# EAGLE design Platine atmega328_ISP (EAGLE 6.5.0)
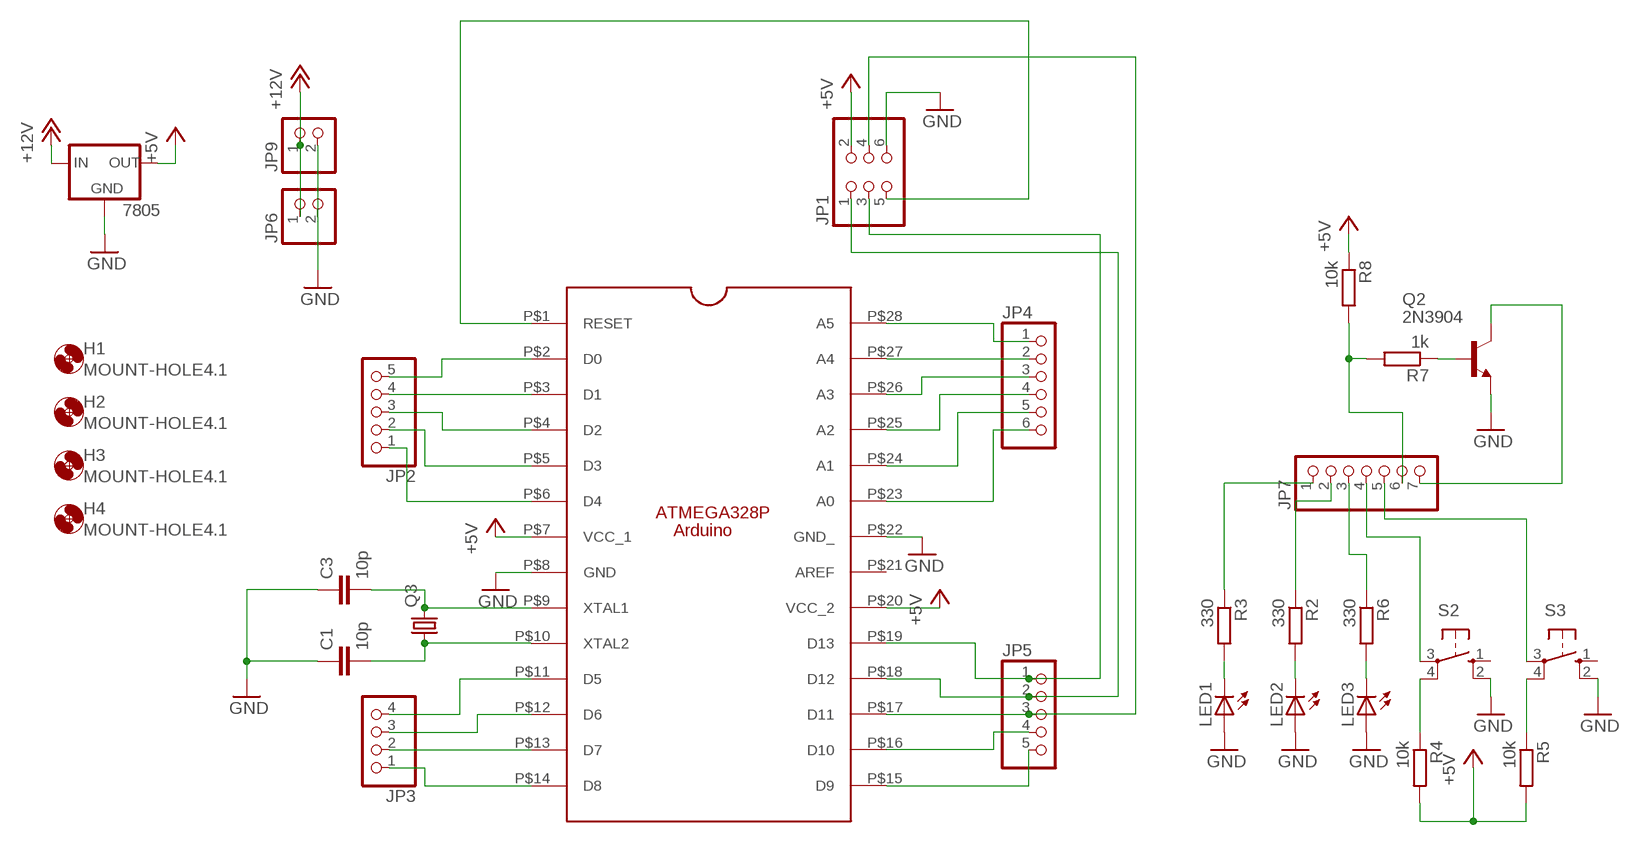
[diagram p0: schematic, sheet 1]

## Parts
7805  78LXX  [78LXX]
C1  10p  C-EU050-025X075  [C050-025X075]
C3  10p  C-EU050-025X075  [C050-025X075]
H1  MOUNT-HOLE4.1  [4,1]
H2  MOUNT-HOLE4.1  [4,1]
H3  MOUNT-HOLE4.1  [4,1]
H4  MOUNT-HOLE4.1  [4,1]
JP1  PINHD-2X3/OCT  [2X03]
JP2  PINHD-1X5  [1X05]
JP3  PINHD-1X4  [1X04]
JP4  PINHD-1X6  [1X06]
JP5  PINHD-1X5  [1X05]
JP6  PINHD-1X2  [1X02]
JP7  PINHD-1X7  [1X07]
JP9  PINHD-1X2  [1X02]
LED1  LED3MM  [LED3MM]
LED2  LED3MM  [LED3MM]
LED3  LED3MM  [LED3MM]
Q2  2N3904  [TO92]
Q3  CRYSTALHC49S  [HC49/S]
R2  330  R-EU_0207/7  [0207/7]
R3  330  R-EU_0207/7  [0207/7]
R4  10k  R-EU_0207/7  [0207/7]
R5  10k  R-EU_0207/7  [0207/7]
R6  330  R-EU_0207/7  [0207/7]
R7  1k  R-EU_0207/7  [0207/7]
R8  10k  R-EU_0207/7  [0207/7]
S2  10-XX  [B3F-10XX]
S3  10-XX  [B3F-10XX]
U1  ATMEGA328P  [ATMEGA328P]

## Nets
7805: 7805.OUT ; supply symbol labelled +5V
+5V: JP1.2 R4.2 R5.2 R8.1 U1.P$7(VCC_1) U1.P$20(VCC_2)
+12V: 7805.IN JP6.1 JP9.1
GND: 7805.GND C1.1 C3.1 JP1.6 JP9.2 LED1.A LED2.A LED3.A Q2.3(E) S2.2(S1) S3.2(S1) U1.P$8(GND) U1.P$22(GND_)
N$1: C3.2 Q3.2 U1.P$9(XTAL1)
N$2: C1.2 Q3.1 U1.P$10(XTAL2)
N$3: JP1.5 U1.P$1(RESET)
N$4: JP2.5 U1.P$2(D0)
N$5: JP2.4 U1.P$3(D1)
N$6: JP2.3 U1.P$4(D2)
N$7: JP2.2 U1.P$5(D3)
N$8: JP2.1 U1.P$6(D4)
N$9: JP5.5 U1.P$15(D9)
N$10: JP5.4 U1.P$16(D10)
N$11: JP1.4 JP5.3 U1.P$17(D11)
N$12: JP1.1 JP5.2 U1.P$18(D12)
N$13: JP1.3 JP5.1 U1.P$19(D13)
N$14: JP4.1 U1.P$28(A5)
N$15: JP4.2 U1.P$27(A4)
N$16: JP4.3 U1.P$26(A3)
N$17: JP4.4 U1.P$25(A2)
N$18: JP4.5 U1.P$24(A1)
N$19: JP4.6 U1.P$23(A0)
N$20: LED1.K(C) R3.2
N$21: R4.1 S2.4(P1)
N$22: JP7.7 Q2.1(C)
N$23: R5.1 S3.4(P1)
N$24: JP7.1 R3.1
N$25: LED2.K(C) R2.2
N$26: LED3.K(C) R6.2
N$27: JP7.2 R2.1
N$28: JP7.3 R6.1
N$29: JP7.4 S2.3(P)
N$30: JP7.5 S3.3(P)
N$31: JP7.6 R7.2 R8.2
N$32: Q2.2(B) R7.1
N$33: JP3.1 U1.P$14(D8)
N$34: JP3.2 U1.P$13(D7)
N$35: JP3.3 U1.P$12(D6)
N$36: JP3.4 U1.P$11(D5)
Unconnected: JP6.2 S2.1(S) S3.1(S) U1.P$21(AREF)

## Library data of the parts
7805 = v-reg:78LXX: VOLTAGE REGULATOR
C1 C3 = rcl:C-EU: CAPACITOR, European symbol
H1-H4 = holes:MOUNT-HOLE: MOUNTING HOLE with drill center marker
JP1 = pinhead_v2:PINHD-2X3: PIN HEADER
JP2 JP5 = pinhead:PINHD-1X5: PIN HEADER
JP3 = pinhead:PINHD-1X4: PIN HEADER
JP4 = pinhead:PINHD-1X6: PIN HEADER
JP6 JP9 = pinhead:PINHD-1X2: PIN HEADER
JP7 = pinhead:PINHD-1X7: PIN HEADER
LED1-LED3 = led:LED: LED
Q2 = transistor-npn:2N3904: NPN Transistor
Q3 = crystal:CRYSTAL: CRYSTAL
R2-R8 = rcl:R-EU_: RESISTOR, European symbol
S2 S3 = switch-omron:10-XX: OMRON SWITCH; MPN: B3F-1000; OC_FARNELL: 176432; OC_NEWARK: 36M3542
U1 = Atmega328P:ATMEGA328P

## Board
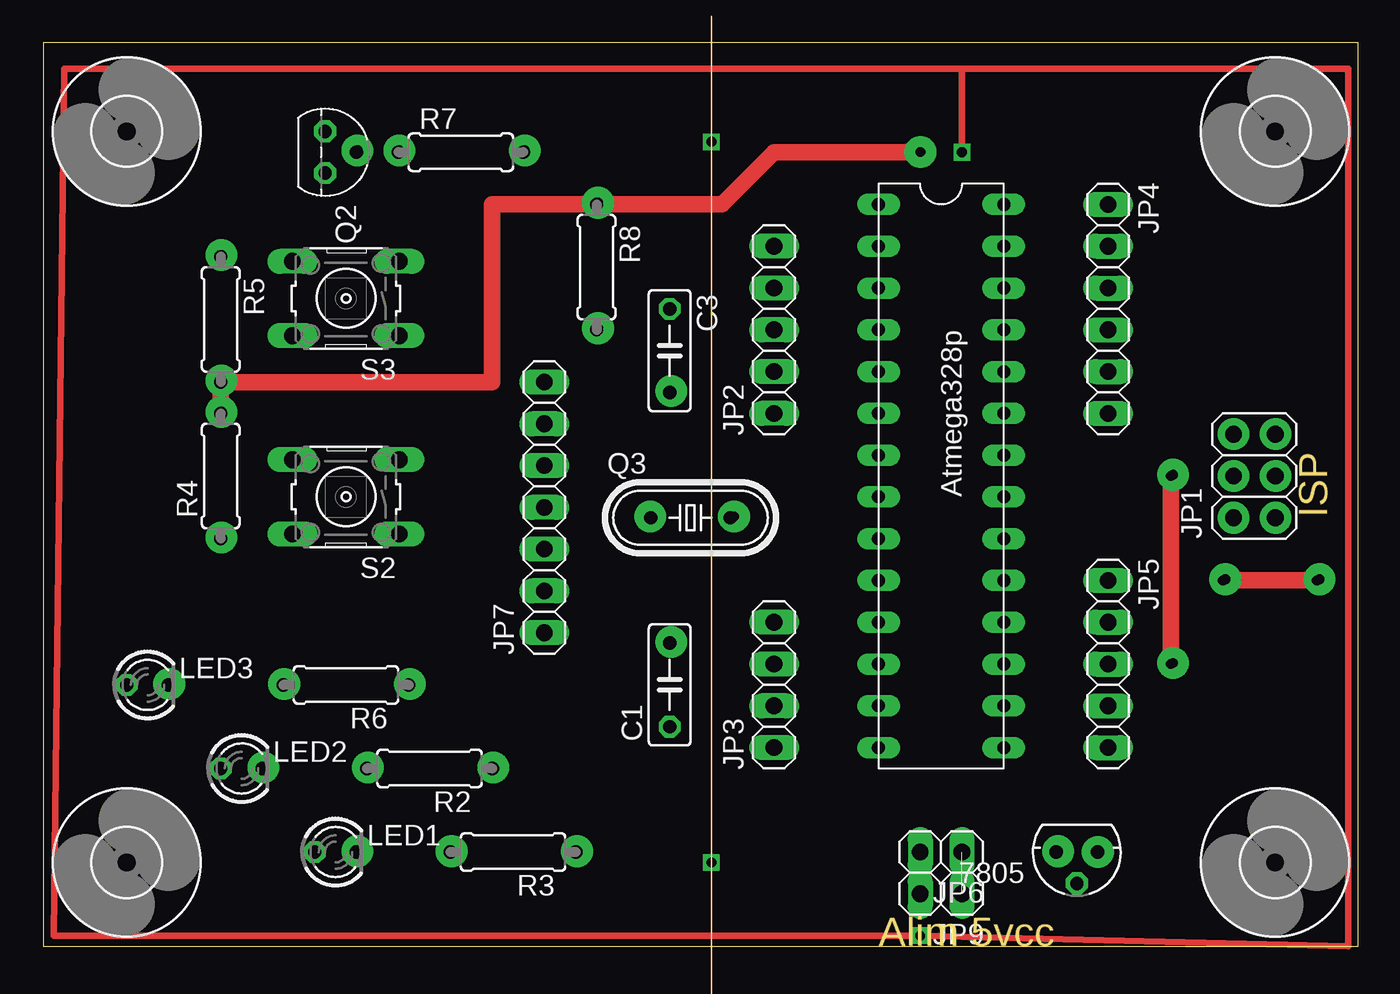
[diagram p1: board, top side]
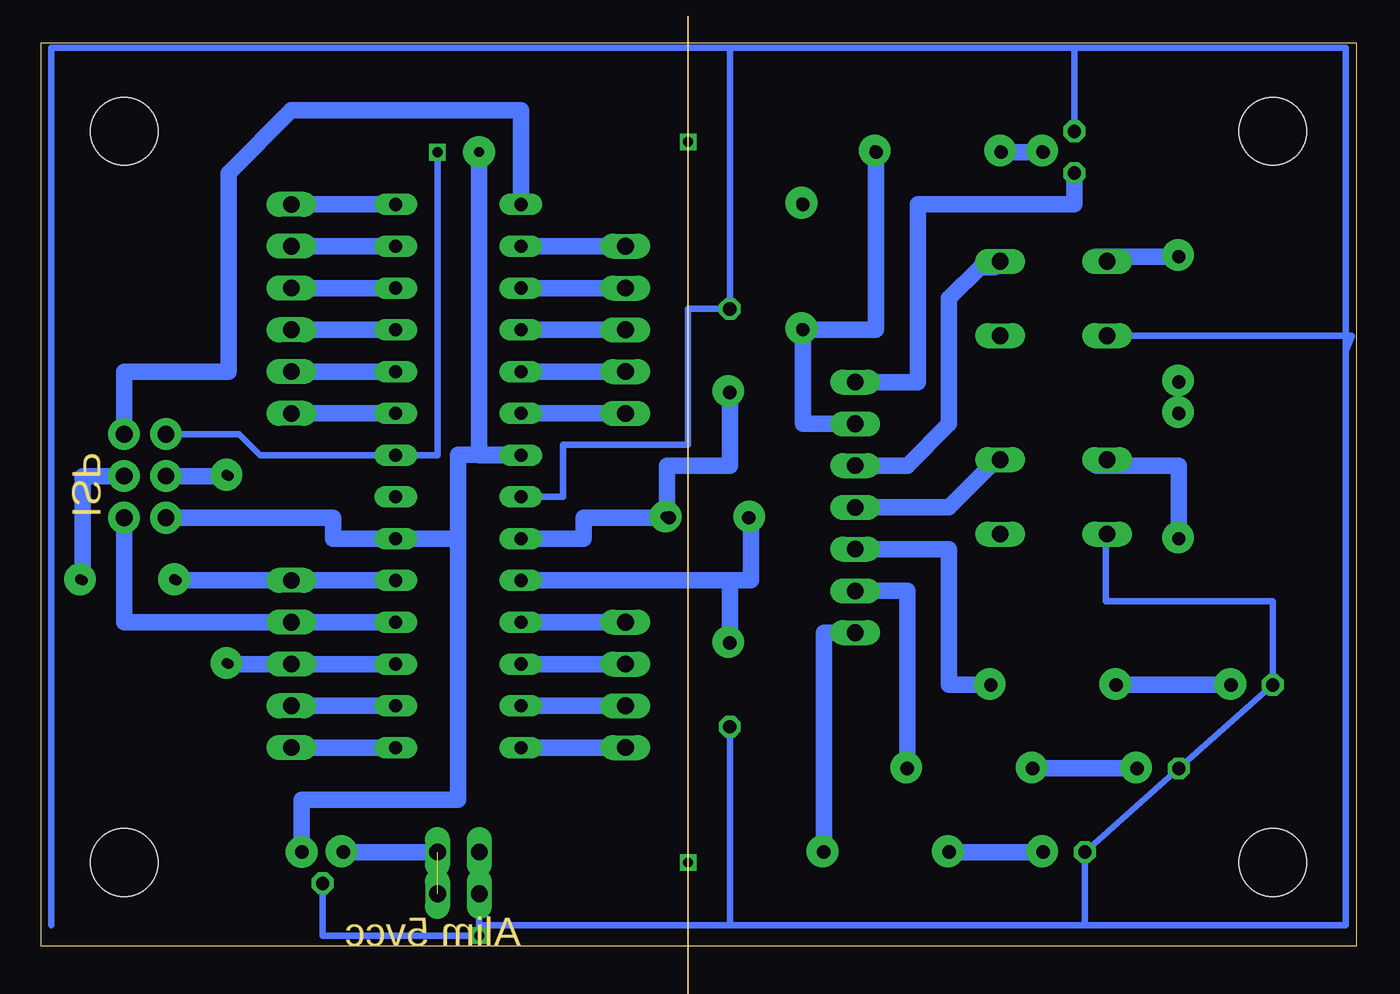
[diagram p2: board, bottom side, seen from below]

Size 79.99 x 54.91 mm. Coordinates in mm from the lower left corner, seen from the top.
Outline: 0,0 79.99,0 79.99,54.91 0,54.91 0,0
Copper layers (1*16): Top 0.035mm / dielectric 1.5mm / Bottom 0.035mm
Design rules "default": minimum track width 10mil, minimum drill 24mil, track to track 8mil, track to pad 8mil, pad to pad 8mil, via to via 8mil, smd to smd 8mil, copper to edge 40mil, drill to drill 8mil, minimum pad ring 10mil, minimum via ring 8mil, stop-mask expansion 4mil, vias tented up to drill 0mil, thermal gap 10mil
Milling: 1 lines

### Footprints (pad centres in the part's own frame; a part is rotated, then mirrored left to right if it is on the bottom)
78LXX = drill 0.813 octagon: GND 0,1.905; IN 1.27,0; OUT -1.27,0
C050-025X075 = drill 0.813 octagon: 1 -2.54,0; 2 2.54,0
4,1 = hole 4.1: 0,0
2X03 = drill 1.016 octagon: 1 -2.54,-1.27; 2 -2.54,1.27; 3 0,-1.27; 4 0,1.27; 5 2.54,-1.27; 6 2.54,1.27
1X05 = drill 1.016 long: 1 -5.08,0; 2 -2.54,0; 3 0,0; 4 2.54,0; 5 5.08,0
1X04 = drill 1.016 long: 1 -3.81,0; 2 -1.27,0; 3 1.27,0; 4 3.81,0
1X06 = drill 1.016 long: 1 -6.35,0; 2 -3.81,0; 3 -1.27,0; 4 1.27,0; 5 3.81,0; 6 6.35,0
1X02 = drill 1.016 long: 1 -1.27,0; 2 1.27,0
1X07 = drill 1.016 long: 1 -7.62,0; 2 -5.08,0; 3 -2.54,0; 4 0,0; 5 2.54,0; 6 5.08,0; 7 7.62,0
LED3MM = drill 0.813 octagon: A -1.27,0; K 1.27,0
TO92 = drill 0.813 octagon: 1 1.27,0; 2 0,1.905; 3 -1.27,0
HC49/S = drill 0.813: 1 -2.413,0; 2 2.413,0
0207/7 = drill 0.813 octagon: 1 -3.81,0; 2 3.81,0
B3F-10XX = drill 1.016 long: 1 -3.251,2.261; 2 3.251,2.261; 3 -3.251,-2.261; 4 3.251,-2.261
ATMEGA328P = drill 0.8 long: P$1 -3.81,15.24; P$2 -3.81,12.7; P$3 -3.81,10.16; P$4 -3.81,7.62; P$5 -3.81,5.08; P$6 -3.81,2.54; P$7 -3.81,0; P$8 -3.81,-2.54; P$9 -3.81,-5.08; P$10 -3.81,-7.62; P$11 -3.81,-10.16; P$12 -3.81,-12.7; P$13 -3.81,-15.24; P$14 -3.81,-17.78; P$15 3.81,-17.78; P$16 3.81,-15.24; P$17 3.81,-12.7; P$18 3.81,-10.16; P$19 3.81,-7.62; P$20 3.81,-5.08; P$21 3.81,-2.54; P$22 3.81,0; P$23 3.81,2.54; P$24 3.81,5.08; P$25 3.81,7.62; P$26 3.81,10.16; P$27 3.81,12.7; P$28 3.81,15.24

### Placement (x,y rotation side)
7805  62.86,5.71 180 top
C1  38.1,15.87 90 top
C3  38.1,36.19 270 top
H1  74.93,5.08 0 top
H2  74.93,49.53 0 top
H3  5.08,5.08 0 top
H4  5.08,49.53 0 top
JP1  73.66,28.57 90 top
JP2  44.45,37.47 90 top
JP3  44.45,15.87 90 top
JP4  64.77,38.73 270 top
JP5  64.77,17.14 270 top
JP6  54.61,5.71 180 top
JP7  30.48,26.67 90 top
JP9  54.61,3.18 180 top
LED1  17.78,5.71 0 top
LED2  12.07,10.79 0 top
LED3  6.35,15.87 0 top
Q2  17.14,48.26 270 top
Q3  39.37,26.04 0 top
R2  23.5,10.79 180 top
R3  28.57,5.71 180 top
R4  10.79,28.57 90 top
R5  10.79,38.1 270 top
R6  18.42,15.87 180 top
R7  25.4,48.26 0 top
R8  33.66,41.27 270 top
S2  18.42,27.3 180 top
S3  18.42,39.37 180 top
U1  54.61,29.85 0 top

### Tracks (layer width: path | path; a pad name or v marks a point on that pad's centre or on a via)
+5V  (via drill 0.6 pad 1.93)
  Top 1.016: R4.2 R5.2 27.31,34.29 27.31,45.1 R8.1 41.27,45.08 44.46,48.27 v53.35,48.27
  Bottom 1.016: JP1.2 62.23,26.04 62.23,24.76 U1.P$20 54.62,24.76 | 54.62,24.76 54.62,8.89 64.15,8.89 64.15,5.72 | 54.62,24.76 54.62,29.85 U1.P$7 53.35,29.85 v53.35,48.27
+12V  (1 unrouted)
  Bottom 1.016: 7805.IN JP6.1
GND  (via drill 0.6)
  Top 0.406: v55.88,48.26 55.88,53.34 | 55.88,53.34 79.38,53.34 79.38,0 v53.34,0.63 0.64,0.63 1.27,53.34 55.88,53.34
  Bottom 0.406: 38.1,54.61 C3.1 40.64,38.73 40.64,30.48 48.26,30.48 48.26,27.3 U1.P$8 | 38.1,54.61 79.38,54.61 79.38,1.27 | 53.34,1.27 38.1,1.27 | 38.1,1.27 16.51,1.27 | 16.51,1.27 0.64,1.27 0.64,36.19 | 0.64,36.19 0.64,54.61 17.14,54.61 | 17.14,54.61 38.1,54.61 | C1.1 38.1,1.27 | v55.88,48.26 55.88,29.85 U1.P$22 66.67,29.85 67.94,31.11 JP1.6 | S3.2 0.28,37.11 0.64,36.19 | 16.51,1.27 LED1.A LED2.A LED3.A 5.08,20.96 15.24,20.96 15.24,24.97 S2.2 | Q2.3 17.14,54.61 | 53.34,6.98 JP9.2 53.34,1.27 | 53.34,1.27 v53.34,0.63 62.86,0.63 7805.GND
N$1
  Bottom 1.016: C3.2 38.1,29.21 41.91,29.21 41.91,26.16 Q3.2 46.99,26.04 46.99,24.76 U1.P$9
N$2
  Bottom 1.016: U1.P$10 38.1,22.22 | 38.1,22.22 36.83,22.22 36.83,25.91 Q3.1 | C1.2 38.1,22.22
N$3
  Bottom 1.016: U1.P$1 50.8,50.8 64.77,50.8 68.58,46.99 68.58,34.92 74.93,34.92 JP1.5
N$4
  Bottom 1.016: JP2.5 U1.P$2
N$5
  Bottom 1.016: JP2.4 U1.P$3
N$6
  Bottom 1.016: JP2.3 U1.P$4
N$7
  Bottom 1.016: JP2.2 U1.P$5
N$8
  Bottom 1.016: JP2.1 U1.P$6
N$9
  Bottom 1.016: U1.P$15 JP5.5
N$10
  Bottom 1.016: U1.P$16 JP5.4
N$11  (via drill 0.6)
  Top 1.016: v68.58,17.14 v68.58,28.57
  Bottom 1.016: U1.P$17 JP5.3 v68.58,17.14 | v68.58,28.57 JP1.4
N$12
  Bottom 1.016: U1.P$18 JP5.2 74.93,19.68 JP1.1
N$13  (via drill 0.6)
  Top 1.016: v71.75,22.22 v77.47,22.22
  Bottom 1.016: U1.P$19 JP5.1 v71.75,22.22 | v77.47,22.22 77.47,28.57 JP1.3
N$14
  Bottom 1.016: U1.P$28 JP4.1
N$15
  Bottom 1.016: U1.P$27 JP4.2
N$16
  Bottom 1.016: U1.P$26 JP4.3
N$17
  Bottom 1.016: JP4.4 U1.P$25
N$18
  Bottom 1.016: U1.P$24 JP4.5
N$19
  Bottom 1.016: U1.P$23 JP4.6
N$20
  Bottom 1.016: LED1.K R3.2
N$21
  Bottom 1.016: R4.1 10.79,29.21 15.8,29.21 S2.4
N$22
  Bottom 1.016: JP7.7 26.67,34.29 26.67,45.08 17.14,45.08 Q2.1
N$23
  Bottom 1.016: R5.1 15.8,41.91 S3.4
N$24
  Bottom 1.016: 29.85,19.05 JP7.1 32.39,19.05 R3.1
N$25
  Bottom 1.016: LED2.K R2.2
N$26
  Bottom 1.016: LED3.K R6.2
N$27
  Bottom 1.016: JP7.2 27.31,21.59 R2.1
N$28
  Bottom 1.016: JP7.3 24.76,24.13 24.76,15.87 R6.1
N$29
  Bottom 1.016: JP7.4 24.76,26.67 22.3,29.13 22.3,29.21 S2.3
N$30
  Bottom 1.016: JP7.5 27.31,29.21 24.76,31.75 24.76,39.37 22.86,41.27 22.02,41.27 S3.3
N$31
  Bottom 1.016: JP7.6 33.66,31.75 R8.2 29.21,37.47 R7.2
N$32
  Bottom 1.016: Q2.2 R7.1
N$33
  Bottom 1.016: JP3.1 U1.P$14
N$34
  Bottom 1.016: U1.P$13 JP3.2
N$35
  Bottom 1.016: JP3.3 U1.P$12
N$36
  Bottom 1.016: JP3.4 U1.P$11
N$37  (via drill 0.6)
  other vias: 40.64,48.89
N$38  (via drill 0.6)
  other vias: 40.64,5.08
N$39  (via drill 0.6 pad 1.93)
  other vias: 29.29,48.37
N$40  (via drill 0.6 pad 1.93)
  other vias: 21.66,48.37
N$41  (via drill 0.6 pad 1.93)
  other vias: 10.85,42.01
N$42  (via drill 0.6 pad 1.93)
  other vias: 10.85,34.38
N$43  (via drill 0.6 pad 1.93)
  other vias: 10.85,32.47
N$44  (via drill 0.6 pad 1.93)
  other vias: 10.85,24.84
N$45  (via drill 0.6 pad 1.93)
  other vias: 7.67,15.94
N$46  (via drill 0.6 pad 1.93)
  other vias: 13.39,10.85
N$47  (via drill 0.6 pad 1.93)
  other vias: 19.11,5.76
N$48  (via drill 0.6 pad 1.93)
  other vias: 14.66,15.94
N$49  (via drill 0.6 pad 1.93)
  other vias: 22.29,15.94
N$50  (via drill 0.6 pad 1.93)
  other vias: 19.75,10.85
N$51  (via drill 0.6 pad 1.93)
  other vias: 27.38,10.85
N$52  (via drill 0.6 pad 1.93)
  other vias: 24.84,5.76
N$53  (via drill 0.6 pad 1.93)
  other vias: 32.47,5.76
N$54  (via drill 0.6 pad 1.93)
  other vias: 38.19,18.48
N$55  (via drill 0.6 pad 1.93)
  other vias: 38.19,33.75
N$56  (via drill 0.6 pad 1.93)
  other vias: 36.92,26.11
N$57  (via drill 0.6 pad 1.93)
  other vias: 42.01,26.11
N$58  (via drill 0.6 pad 1.93)
  other vias: 33.74,45.19
N$59  (via drill 0.6 pad 1.93)
  other vias: 33.74,37.56
N$60  (via drill 0.6 pad 1.93)
  other vias: 68.72,28.65
N$61  (via drill 0.6 pad 1.93)
  other vias: 68.72,17.21
N$62  (via drill 0.6 pad 1.93)
  other vias: 71.9,22.3
N$63  (via drill 0.6 pad 1.93)
  other vias: 77.63,22.3
N$64  (via drill 0.6 pad 1.93)
  other vias: 61.73,5.76
N$65  (via drill 0.6 pad 1.93)
  other vias: 19.11,48.37
N$66  (via drill 0.6 pad 1.93)
  other vias: 72.4,31.12
N$67  (via drill 0.6 pad 1.93)
  other vias: 74.95,31.12
N$68  (via drill 0.6 pad 1.93)
  other vias: 74.95,28.58
N$69  (via drill 0.6 pad 1.93)
  other vias: 72.4,28.58
N$70  (via drill 0.6 pad 1.93)
  other vias: 72.4,26.04
N$71  (via drill 0.6 pad 1.93)
  other vias: 74.95,26.04
N$72  (via drill 0.6 pad 1.93)
  other vias: 64.15,5.72

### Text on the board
Milling: Platine ATMEGA328_ISP | ISP | Alim 5vcc | Centrage CNC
